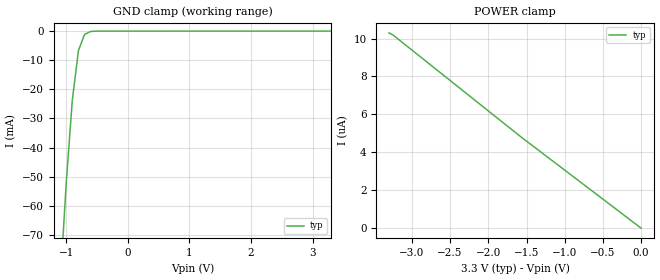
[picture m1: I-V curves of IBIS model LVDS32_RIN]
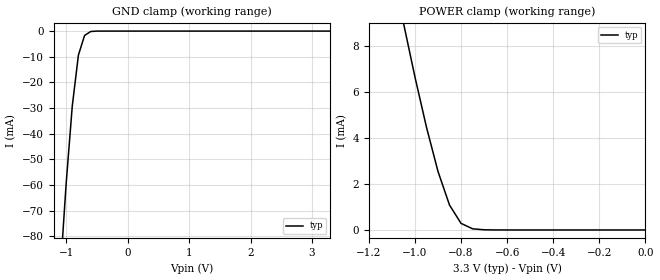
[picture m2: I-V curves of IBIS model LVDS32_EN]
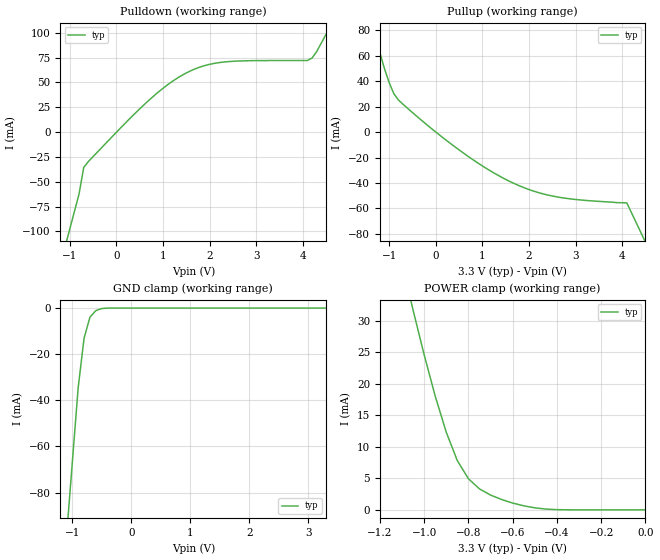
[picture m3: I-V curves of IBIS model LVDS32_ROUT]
|   Texas Instruments Incorporated
|   Data Transmissions Products
|   IBIS Model for SN65LVDS32
|   16W  Package
[IBIS Ver]   2.1
[Comment char]   |_char
[File name]   lvds32w.ibs
[File Rev]   2.0
[Date]   25Jul97 | Updated May 2009 for Ceramic W parasitics
[Source]   File originated at Texas Instruments Incorporated.
   Data Transmission Products Group. All data based on
   Bench Measurements.
[Notes]
[Disclaimer]
(C) Copyright Texas Instruments Incorporated 1997
   All rights reserved
  Texas Instruments Incorporated hereby grants the user of this IBIS
model a non-exclusive, nontransferable license to use this IBIS model
under the following terms.  Before using this IBIS model, the user
should read this license.  If the user does not accept these terms,
the IBIS model should be returned to Texas Instruments within 30 days.
  The user is granted this license only to use the IBIS model and
is not granted rights to sell, load, rent, lease or license the IBIS
model in whole or in part, or in modified form to anyone other than
user.  User may modify the IBIS model to suit its specific applications
but rights to derivative works and such modifications shall belong to
Texas Instruments.
  This IBIS model is provided on an "AS IS" basis and Texas Instruments
makes absolutely no warranty with respect to the information contained
herein.  TEXAS INSTRUMENTS DISCLAIMS AND CUSTOMER WAIVES ALL WARRANTIES,
EXPRESS OR IMPLIED, INCLUDING WARRANTIES OF MERCHANTABILITY OR FITNESS
FOR A PARTICULAR PURPOSE. The entire risk as to quality and performance
is with the Customer. ACCORDINGLY, IN NO EVENT SHALL THE COMPANY BE LIABLE
FOR ANY DAMAGES, WHETHER IN CONTRACT OR TORT,INCLUDING ANY LOST PROFITS
OR OTHER INCIDENTAL, CONSEQUENTIAL, EXEMPLARY, OR PUNITIVE DAMAGES ARISING
OUT OF THE USE OR APPLICATION OF THE IBIS model provided in this package.
Further, Texas Instruments reserves the right to discontinue or make changes
without notice to any product herein to improve reliability, function, or
design. Texas Instruments does not convey any license under patent rights
or any other intellectual property rights, including those of third parties.
Contact Texas Instruments at ATTN:DATA TRANSMISSIONS
Thomas Fisher 8505 Forest Lane, M/S 8710, Dallas, TX 75243-4136
[Copyright]   Copyright 1997, Texas Instruments, All Rights Reserved
[Component]   SN55LVDS32W
[Manufacturer]  Texas Instruments Incorporated
[Package]
|   typ   min   max
R_pkg   0.177   0.141   0.245
L_pkg   3.230nH   2.617nH   4.412nH
C_pkg   1.228pF   1.057pF   1.531pF
[Pin]   signal_name   model_name   R_pin   L_pin   C_pin
1   1B   LVDS32_RIN   0.244   4.385n   1.524p
2   1A   LVDS32_RIN   0.176   3.183n   1.235p
3   1Y   LVDS32_ROUT   0.142   2.637n   1.071p
4   G   LVDS32_EN   0.144   2.645n   1.060p
5   2Y   LVDS32_ROUT   0.147   2.708n   1.081p
6   2A   LVDS32_RIN   0.144   2.687n   1.092p
7   2B   LVDS32_RIN   0.176   3.182n   1.236p
8   GND   GND   0.245   4.412n   1.531p
9   3B   LVDS32_RIN   0.245   4.411n   1.531p
10   3A   LVDS32_RIN   0.176   3.183n   1.235p
11   3Y   LVDS32_ROUT   0.141   2.619n   1.064p
12   /G   LVDS32_EN   0.144   2.639n   1.057p
13   4Y   LVDS32_ROUT   0.150   2.772n   1.102p
14   4A   LVDS32_RIN   0.141   2.617n   1.063p
15   4B   LVDS32_RIN   0.176   3.182n   1.235p
16   VCC   POWER   0.245   4.411n   1.531p
[Diff_pin]   inv_pin   vdiff   tdelay_typ   tdelay_min   tdelay_max
| The 'xA' pin is Diff_pin and the 'xB' pin is the inv_pin
2   1   100mV   0 0 0   | Vth  +/-100mV
6   7   100mV   0 0 0
10   9   100mV   0 0 0
14   15   100mV   0 0 0
| Models and submodels in the file (3): LVDS32_RIN (Input), LVDS32_EN (Input), LVDS32_ROUT (3-state)
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|   Receiver Input  MODEL
[Model]   LVDS32_RIN
Model_type   Input
|Signals   1A,1B,2A,2B,3A,3B,4A,4B
Vinh = 2.0
Vinl = 0.8
|   typ   min   max
C_comp   1.0pF   NA   NA
|   typ   min   max
[Temperature Range]   25.0   NA   NA
[Voltage range]   3.3V   3.0V   3.6V
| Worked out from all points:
|   GND clamp passes 1 mA (typ) near -0.69 V on its own axis
[GND_clamp]
|   Voltage   I(typ)   I(min)   I(max)
-3.3V     -873.9mA   NA         NA
-1.1V     -88.23mA   NA         NA
-1V       -52.52mA   NA         NA
-900mV    -23.67mA   NA         NA
-800mV    -6.59mA    NA         NA
-700mV    -1.12mA    NA         NA
-600mV    -120uA     NA         NA
-500mV    -15.1uA    NA         NA
3.3V      474pA      NA         NA
[Power_clamp]
| Note that the[POWER_clamp]voltage table is referenced to Vcc
| and is calculated using Vtable=Vcc - Vmeasured.
|   Voltage   I(typ)   I(min)   I(max)
-3.3V     10.3uA     NA         NA
-3.25V    10.2uA     NA         NA
-1.55V    4.74uA     NA         NA
-1.5V     4.59uA     NA         NA
-50mV     149nA      NA         NA
0V        -3.35nA    NA         NA
|   Receiver Enable  MODEL
[Model]   LVDS32_EN
Model_type   Input
|Signals   G,/G
Vinh = 2.0
Vinl = 0.8
|   typ   min   max
C_comp   1.0pF   NA   NA
|   typ   min   max
[Temperature Range]   25.0   NA   NA
[Voltage range]   3.3V   3.0V   3.6V
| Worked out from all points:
|   GND clamp passes 1 mA (typ) near -0.65 V on its own axis
|   POWER clamp passes 1 mA (typ) near -0.84 V on its own axis
[GND_clamp]
|   Voltage   I(typ)   I(min)   I(max)
-3.3V     -895.7mA   NA         NA
-1.1V     -95.97mA   NA         NA
-1V       -59.62mA   NA         NA
-900mV    -29.24mA   NA         NA
-800mV    -9.37mA    NA         NA
-700mV    -1.72mA    NA         NA
-600mV    -160uA     NA         NA
-500mV    -4.9uA     NA         NA
-400mV    -110nA     NA         NA
3.3V      3.96nA     NA         NA
[Power_clamp]
| Note that the[POWER_clamp]voltage table is referenced to Vcc
| and is calculated using Vtable=Vcc - Vmeasured.
|   Voltage   I(typ)   I(min)   I(max)
-3.3V     142mA      NA         NA
-1.05V    8.99mA     NA         NA
-1V       6.64mA     NA         NA
-950mV    4.46mA     NA         NA
-900mV    2.54mA     NA         NA
-850mV    1.08mA     NA         NA
-800mV    286uA      NA         NA
-750mV    51uA       NA         NA
-700mV    7.83uA     NA         NA
0V        1.77nA     NA         NA
|   Receiver Output  MODEL
[Model]   LVDS32_ROUT
Model_type   3-state
| Signals   1Y,2Y,3Y,4Y
Vmeas = 1.5V   |Reference voltage for timing measurements
Cref = 8pF   |Timing specification test load capacitance value
Vref = 0   |Timing specification test load voltage; GND
| variable   typ   min   max
C_comp   1.0pF   NA   NA
|   typ   min   max
[Temperature Range]   25.0   NA   NA
[Voltage range]   3.3V   3.0V   3.6V
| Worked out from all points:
|   slope of the pulldown table from 0 to 0.495 V, typ, clamps not added: 21.2 ohm
|   slope of the pullup table from 0 to 0.495 V, typ, clamps not added: 35.5 ohm
|   GND clamp passes 1 mA (typ) near -0.59 V on its own axis
|   POWER clamp passes 1 mA (typ) near -0.59 V on its own axis
[Pulldown]
|   Voltage   I(typ)   I(min)   I(max)
-3.3V     -505.4mA   NA         NA
-900mV    -79.93mA   NA         NA
-800mV    -62.2mA    NA         NA
-700mV    -35.56mA   NA         NA
-600mV    -29.67mA   NA         NA
800mV     36.29mA    NA         NA
1.6V      61.86mA    NA         NA
2.4V      70.98mA    NA         NA
4.1V      72.09mA    NA         NA
4.2V      74.6mA     NA         NA
4.4V      89.79mA    NA         NA
6.6V      279.1mA    NA         NA
[Pullup]
|   Voltage   I(typ)   I(min)   I(max)
| Note that the[Pullup]voltage table is referenced to Vcc
| and is calculated using Vtable=Vcc - Vmeasured.
-3.3V     394.8mA    NA         NA
-1.4V     92.99mA    NA         NA
-1.3V     77.11mA    NA         NA
-1.2V     62.52mA    NA         NA
-1V       38.96mA    NA         NA
-800mV    25.22mA    NA         NA
600mV     -16.65mA   NA         NA
1.7V      -40.76mA   NA         NA
2.6V      -51.01mA   NA         NA
4.1V      -55.7mA    NA         NA
4.2V      -63.43mA   NA         NA
6.6V      -249mA     NA         NA
| Output in High Impedance (off)
[GND_clamp]
|   Voltage   I(typ)   I(min)   I(max)
-3.3V     -818.5mA   NA         NA
-1.1V     -99.97mA   NA         NA
-1V       -67.31mA   NA         NA
-900mV    -34.61mA   NA         NA
-800mV    -13.09mA   NA         NA
-700mV    -3.91mA    NA         NA
-600mV    -1.1mA     NA         NA
-500mV    -200uA     NA         NA
-400mV    -12.1uA    NA         NA
3.3V      797pA      NA         NA
[POWER_clamp]
|   Voltage   I(typ)   I(min)   I(max)
| Note that the [POWER_clamp] voltage table is referenced to Vcc
| and is calculated using Vtable = Vcc - Vmeasured.
| Outputs in Tri-state.
-3.3V     412.8mA    NA         NA
-1.1V     39.15mA    NA         NA
-1.05V    31.72mA    NA         NA
-1V       24.63mA    NA         NA
-950mV    18.07mA    NA         NA
-900mV    12.32mA    NA         NA
-850mV    7.816mA    NA         NA
-800mV    4.946mA    NA         NA
-750mV    3.33mA     NA         NA
-650mV    1.642mA    NA         NA
-500mV    320uA      NA         NA
0V        803pA      NA         NA
[Ramp]
|   typ   min   max
dV/dt_r   2.0v/512ps   NA   NA
dV/dt_f   2.0v/385ps   NA   NA
R_load = 1MOhm   | Represents an open
